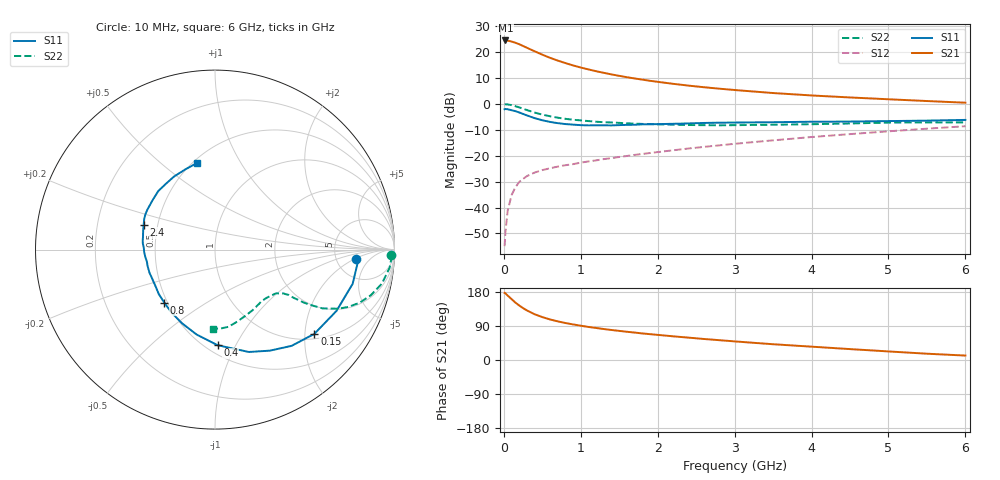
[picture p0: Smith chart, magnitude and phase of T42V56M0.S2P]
! Infineon Technologies  Discrete & RF Semiconductors
! BFR182T
! Si NPN RF Bipolar Junction Transistor in SC75
! VCE = 2.5 V  IC = 6 mA
! Common Emitter S-Parameters:  October  1999
# GHz  S  MA  R  50
!  f  S11  S21  S12  S22
! GHz  MAG  ANG  MAG  ANG  MAG  ANG  MAG  ANG
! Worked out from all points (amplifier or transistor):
!   36 points, 10 MHz to 6 GHz, reference 50 ohm
!   highest |S21| = 24.5 dB at 20 MHz (marker M1)
!   |S21| within 3 dB of that: start of sweep to 313.2 MHz
!   unconditionally stable (mu >= 1): 1.278 GHz to 3.934 GHz
!   at 250 MHz: K = 0.32, MSG = 25.6 dB, |S12| = -28.9 dB
!   at 1.4 GHz: K = 1.04, MAG = 15.0 dB, |S12| = -20.9 dB
!   at 6 GHz: K = 0.84, MSG = 4.5 dB, |S12| = -8.6 dB
!   lowest NFmin = 1.25 dB at 450 MHz
!   S11 on the Smith chart (normalised r, x): 10 MHz: 7.83, -2.22; 150 MHz: 1.13, -2.24; 400 MHz: 0.57, -0.85; 800 MHz: 0.48, -0.34; 2.4 GHz: 0.42, +0.14; 6 GHz: 0.52, +0.67
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0.01  0.7887 -3.9  16.75 177.2  0.0018 81.6  0.9821 -1.9
0.02  0.8005 -4.3  16.8 176.1  0.0033 90.9  0.9851 -2.4
0.05  0.7902 -14.0  16.65 170.0  0.0087 83.0  0.9779 -6.0
0.1  0.7581 -26.8  16 160.7  0.0173 76.7  0.9492 -11.5
0.15  0.7258 -40.3  15.18 151.6  0.0246 71.4  0.9048 -16.3
0.2  0.6853 -51.5  14.21 143.8  0.0312 67.6  0.8582 -20.2
0.25  0.6406 -61.5  13.15 136.9  0.0358 63.0  0.8076 -23.3
0.3  0.6008 -71.7  12.14 130.8  0.0405 60.4  0.7624 -25.6
0.4  0.5327 -88.5  10.38 120.7  0.0474 55.9  0.6821 -28.7
0.5  0.4842 -102.2  8.932 113.3  0.0529 54.0  0.623 -29.9
0.6  0.4499 -114.1  7.766 107.0  0.0573 54.1  0.5786 -30.8
0.7  0.4262 -124.7  6.876 102.0  0.0617 53.7  0.5434 -31.1
0.8  0.4088 -133.7  6.151 97.6  0.0657 54.3  0.5167 -31.5
1.1  0.3856 -155.2  4.634 87.2  0.0777 56.1  0.4669 -32.2
1.4  0.3854 -170.0  3.713 79.2  0.0899 58.0  0.4388 -33.9
1.6  0.3951 -178.3  3.279 74.5  0.099 59.2  0.4228 -35.1
2.2  0.414 165.2  2.447 62.5  0.1275 62.0  0.3986 -41.1
2.4  0.4208 160.8  2.258 59.0  0.138 62.5  0.3923 -43.7
3.5  0.4437 141.5  1.623 41.6  0.1984 62.1  0.3973 -58.2
4.5  0.4572 127.2  1.334 28.8  0.2617 58.9  0.4199 -72.9
5.5  0.4766 110.2  1.138 16.6  0.3332 53.9  0.4409 -86.0
6  0.492 102.0  1.057 11.7  0.3717 50.4  0.44 -91.6
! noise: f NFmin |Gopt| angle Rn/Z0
0.45  1.25  0.25  39  0.3
0.9  1.4  0.25  78  0.23
1.8  1.95  0.21  151  0.2
